| IBIS file stm32u575_585_lqfp100.ibs
[IBIS ver] 4.2
[File name] stm32u575_585_lqfp100.ibs
[File Rev] 1.0
[Date]   06-08-2021
[Source] Data Created at STMicroelectronics
[Notes]  File originated from ELDO simulations.
[Disclaimer]  This information is for modeling purpose only and is
   not guaranted. The information is subject to change without
   notice.
[Copyright] Copyright 2021 STMicroelectronics Inc.
|   Component stm32u575_585_lqfp100
[Component] stm32u575_585_lqfp100
[Manufacturer] STMicroelectronics
[Package]
| variable   typ   min   max
R_pkg   0   NA   NA
L_pkg   0   NA   NA
C_pkg   0   NA   NA
[Pin]   signal_name   model_name   R_pin   L_pin   C_pin   | Comment
1 PE2 io8_100m_hslv_ft 132.430E-3 7.034E-9 135.000E-15
2 PE3 io8_100m_hslv_tamp_ft 133.348E-3 6.765E-9 19.500E-15
3 PE4 io8_100m_hslv_tamp_ft 128.973E-3 6.495E-9 10.400E-15
4 PE5 io8_100m_hslv_tamp_ft 125.345E-3 6.206E-9 5.240E-15
5 PE6 io8_100m_hslv_tamp_ft 120.515E-3 5.991E-9 7.820E-15
6 VBAT POWER 120.471E-3 5.950E-9 6.530E-15
7 PC13 io8_100m_ft_v33 117.881E-3 5.783E-9 6.230E-15
8 PC14-OSC32_IN io8_100m_ft 117.279E-3 5.654E-9 3.110E-15
9 PC15-OSC32_OUT io8_100m_ft 115.548E-3 5.548E-9 1.390E-15
10 VSS GND 114.996E-3 5.434E-9 2.920E-15
11 VDD POWER 112.976E-3 5.296E-9 3.560E-15
12 PH0-OSC_IN io8_100m_ft 111.323E-3 5.231E-9 4.780E-15
13 PH1-OSC_OUT io8_100m_ft 109.217E-3 5.142E-9 8.660E-15
14 NRST nc 110.664E-3 5.180E-9 9.030E-15
15 PC0 io8_100m_hslv_ft 110.608E-3 5.192E-9 7.980E-15
16 PC1 io8_166m_hslv_i2c_ft 111.326E-3 5.252E-9 10.300E-15
17 PC2 io8_100m_hslv_ft 114.420E-3 5.345E-9 7.000E-15
18 PC3 io8_100m_hslv_ft 114.363E-3 5.454E-9 8.650E-15
19 VSSA GND 117.564E-3 5.621E-9 7.825E-15
20 VREF- GND 119.905E-3 5.800E-9 229.000E-18
21 VREF+ POWER 122.312E-3 5.963E-9 1.050E-15
22 VDDA POWER 125.384E-3 6.187E-9 812.000E-18
23 PA0 io8_100m_hslv_tamp_ft 129.702E-3 6.485E-9 3.820E-15
24 PA1 io8_100m_hslv_tamp_ft 132.290E-3 6.715E-9 6.800E-15
25 PA2 io8_100m_hslv_ft 132.955E-3 7.014E-9 16.700E-15
26 PA3 io8_166m_hslv_ft 133.943E-3 7.050E-9 17.500E-15
27 VSS GND 134.958E-3 6.804E-9 12.700E-15
28 VDD POWER 130.511E-3 6.528E-9 9.830E-15
29 PA4 io8_100m_hslv_ft 125.387E-3 6.245E-9 6.070E-15
30 PA5 io8_100m_ft 124.989E-3 6.108E-9 577.000E-18
31 PA6 io8_100m_hslv_ft 121.784E-3 5.890E-9 1.520E-15
32 PA7 io8_100m_hslv_ft 119.149E-3 5.716E-9 5.440E-15
33 PC4 io8_100m_hslv_ft 116.375E-3 5.556E-9 4.100E-15
34 PC5 io8_100m_tamp_ft 113.279E-3 5.415E-9 3.690E-15
35 PB0 io8_100m_hslv_ft 112.727E-3 5.358E-9 3.895E-15
36 PB1 io8_100m_hslv_ft 112.271E-3 5.272E-9 1.660E-15
37 PB2 io8_100m_hslv_tamp_ft 111.816E-3 5.238E-9 7.920E-15
38 PE7 io8_100m_hslv_ft 110.999E-3 5.184E-9 9.900E-15
39 PE8 io8_100m_hslv_ft 114.589E-3 5.299E-9 7.910E-15
40 PE9 io8_166m_hslv_ft 114.461E-3 5.333E-9 7.940E-15
41 PE10 io8_166m_hslv_ft 115.350E-3 5.424E-9 4.180E-15
42 PE11 io8_100m_hslv_ft 116.979E-3 5.533E-9 6.060E-15
43 PE12 io8_100m_hslv_ft 120.185E-3 5.698E-9 5.120E-15
44 PE13 io8_100m_hslv_ft 122.587E-3 5.871E-9 4.740E-15
45 PE14 io8_100m_hslv_ft 126.303E-3 6.069E-9 11.600E-15
46 PE15 io8_100m_hslv_ft 129.715E-3 6.277E-9 9.910E-15
47 PB10 io8_166m_hslv_i2c_ft 133.373E-3 6.508E-9 5.080E-15
48 VCAP POWER 137.888E-3 6.857E-9 5.470E-15
49 VSS GND 131.554E-3 6.802E-9 4.180E-15
50 VDD POWER 132.348E-3 7.042E-9 11.900E-15
51 PB12 io8_166m_hslv_ft 131.768E-3 7.008E-9 16.200E-15
52 PB13 io8_100m_i2c_ft 131.784E-3 6.751E-9 2.150E-15
53 PB14 io8_100m_i2c_ft 129.151E-3 6.483E-9 9.175E-15
54 PB15 nc 125.191E-3 6.202E-9 5.663E-15
55 PD8 io8_100m_hslv_ft 121.530E-3 5.986E-9 3.690E-15
56 PD9 io8_100m_hslv_ft 118.874E-3 5.807E-9 7.430E-15
57 PD10 io8_100m_hslv_ft 115.870E-3 5.635E-9 10.600E-15
58 PD11 io8_100m_hslv_ft 113.226E-3 5.471E-9 5.760E-15
59 PD12 io8_100m_hslv_ft 111.782E-3 5.354E-9 6.530E-15
60 PD13 io8_100m_hslv_ft 110.713E-3 5.276E-9 11.400E-15
61 PD14 io8_100m_hslv_ft 110.052E-3 5.204E-9 13.200E-15
62 PD15 io8_100m_hslv_ft 109.954E-3 5.180E-9 14.600E-15
63 PC6 io8_100m_ft 109.780E-3 5.154E-9 7.250E-15
64 PC7 io8_100m_ft 112.446E-3 5.258E-9 359.000E-18
65 PC8 io8_100m_ft 113.596E-3 5.332E-9 658.000E-18
66 PC9 io8_100m_ft 115.707E-3 5.466E-9 508.500E-18
67 PA8 io8_166m_hslv_ft 116.952E-3 5.598E-9 583.250E-18
68 PA9 io8_100m_usb_vbus_ft 119.043E-3 5.762E-9 545.875E-18
69 PA10 io8_100m_usb_id 120.674E-3 5.880E-9 13.900E-15
70 PA11 io8_usb_ft 124.659E-3 6.108E-9 25.000E-15
71 PA12 io8_usb_ft 124.407E-3 6.161E-9 39.900E-15
72 PA13 io8_100m_ft 130.156E-3 6.404E-9 302.000E-15
73 VDDUSB POWER 135.110E-3 6.824E-9 155.000E-15
74 VSS GND 139.402E-3 7.077E-9 155.000E-15
75 VDD POWER 133.554E-3 7.056E-9 39.000E-15
76 PA14 io8_100m_ft 135.295E-3 7.104E-9 16.300E-15
77 PA15 nc 132.514E-3 6.836E-9 9.760E-15
78 PC10 io8_100m_ft 133.482E-3 6.641E-9 9.300E-15
79 PC11 io8_100m_hslv_ft 128.366E-3 6.341E-9 5.420E-15
80 PC12 io8_166m_hslv_ft 124.282E-3 6.092E-9 1.180E-15
81 PD0 io8_100m_hslv_ft 121.841E-3 5.917E-9 5.460E-15
82 PD1 io8_100m_hslv_ft 118.487E-3 5.728E-9 7.000E-15
83 PD2 io8_100m_ft 117.180E-3 5.573E-9 6.060E-15
84 PD3 io8_166m_hslv_ft 113.501E-3 5.422E-9 5.450E-15
85 PD4 io8_100m_hslv_ft 113.789E-3 5.344E-9 529.000E-18
86 PD5 io8_100m_hslv_ft 110.806E-3 5.256E-9 2.990E-15
87 PD6 io8_166m_hslv_ft 110.442E-3 5.246E-9 2.060E-15
88 PD7 io8_100m_hslv_ft 111.525E-3 5.178E-9 5.680E-15
89 PB3 io8_100m_i2c_ft 111.144E-3 5.223E-9 9.910E-15
90 PB4 io8_100m_i2c_ft 113.222E-3 5.310E-9 9.050E-15
91 PB5 io8_166m_hslv_ft 113.323E-3 5.401E-9 12.900E-15
92 PB6 io8_100m_i2c_ft 115.849E-3 5.519E-9 12.600E-15
93 PB7 io8_166m_hslv_i2c_ft 117.578E-3 5.673E-9 6.140E-15
94 PH3-BOOT0 io8_100m_ft 118.982E-3 5.802E-9 9.370E-15
95 PB8 io8_100m_i2c_ft 121.886E-3 5.962E-9 7.755E-15
96 PB9 io8_100m_i2c_ft 126.276E-3 6.158E-9 8.563E-15
97 PE0 io8_100m_hslv_ft 128.749E-3 6.367E-9 8.159E-15
98 PE1 io8_100m_hslv_ft 133.288E-3 6.700E-9 1.030E-15
99 VSS GND 132.230E-3 6.844E-9 4.410E-15
100 VDD POWER 132.277E-3 7.052E-9 17.100E-15
[Model Selector] io8_100m_ft
io8_100m_ft_hs_1v2  "IO8_FT 100MHz high speed @ 1.2V"
io8_100m_ft_hs_pu_1v2  "IO8_FT 100MHz high speed @ 1.2V pullup"
io8_100m_ft_hs_pd_1v2  "IO8_FT 100MHz high speed @ 1.2V pulldown"
io8_100m_ft_fs_1v2  "IO8_FT 100MHz fast speed @ 1.2V"
io8_100m_ft_fs_pu_1v2  "IO8_FT 100MHz fast speed @ 1.2V pullup"
io8_100m_ft_fs_pd_1v2  "IO8_FT 100MHz fast speed @ 1.2V pulldown"
io8_100m_ft_ms_1v2  "IO8_FT 100MHz med speed @ 1.2V"
io8_100m_ft_ms_pu_1v2  "IO8_FT 100MHz med speed @ 1.2V pullup"
io8_100m_ft_ms_pd_1v2  "IO8_FT 100MHz med speed @ 1.2V pulldown"
io8_100m_ft_ls_1v2  "IO8_FT 100MHz low speed @ 1.2V"
io8_100m_ft_ls_pu_1v2  "IO8_FT 100MHz low speed @ 1.2V pullup"
io8_100m_ft_ls_pd_1v2  "IO8_FT 100MHz low speed @ 1.2V pulldown"
io8_100m_ft_hs_1v8  "IO8_FT 100MHz high speed @ 1.8V"
io8_100m_ft_hs_pu_1v8  "IO8_FT 100MHz high speed @ 1.8V pullup"
io8_100m_ft_hs_pd_1v8  "IO8_FT 100MHz high speed @ 1.8V pulldown"
io8_100m_ft_fs_1v8  "IO8_FT 100MHz fast speed @ 1.8V"
io8_100m_ft_fs_pu_1v8  "IO8_FT 100MHz fast speed @ 1.8V pullup"
io8_100m_ft_fs_pd_1v8  "IO8_FT 100MHz fast speed @ 1.8V pulldown"
io8_100m_ft_ms_1v8  "IO8_FT 100MHz med speed @ 1.8V"
io8_100m_ft_ms_pu_1v8  "IO8_FT 100MHz med speed @ 1.8V pullup"
io8_100m_ft_ms_pd_1v8  "IO8_FT 100MHz med speed @ 1.8V pulldown"
io8_100m_ft_ls_1v8  "IO8_FT 100MHz low speed @ 1.8V"
io8_100m_ft_ls_pu_1v8  "IO8_FT 100MHz low speed @ 1.8V pullup"
io8_100m_ft_ls_pd_1v8  "IO8_FT 100MHz low speed @ 1.8V pulldown"
io8_100m_ft_hs_3v3  "IO8_FT 100MHz high speed @ 3.3V"
io8_100m_ft_hs_pu_3v3  "IO8_FT 100MHz high speed @ 3.3V pullup"
io8_100m_ft_hs_pd_3v3  "IO8_FT 100MHz high speed @ 3.3V pulldown"
io8_100m_ft_fs_3v3  "IO8_FT 100MHz fast speed @ 3.3V"
io8_100m_ft_fs_pu_3v3  "IO8_FT 100MHz fast speed @ 3.3V pullup"
io8_100m_ft_fs_pd_3v3  "IO8_FT 100MHz fast speed @ 3.3V pulldown"
io8_100m_ft_ms_3v3  "IO8_FT 100MHz med speed @ 3.3V"
io8_100m_ft_ms_pu_3v3  "IO8_FT 100MHz med speed @ 3.3V pullup"
io8_100m_ft_ms_pd_3v3  "IO8_FT 100MHz med speed @ 3.3V pulldown"
io8_100m_ft_ls_3v3  "IO8_FT 100MHz low speed @ 3.3V"
io8_100m_ft_ls_pu_3v3  "IO8_FT 100MHz low speed @ 3.3V pullup"
io8_100m_ft_ls_pd_3v3  "IO8_FT 100MHz low speed @ 3.3V pulldown"
[Model Selector] io8_100m_hslv_ft
io8_100m_ft_hs_1v2  "IO8_FT 100MHz high speed @ 1.2V"
io8_100m_ft_hs_pu_1v2  "IO8_FT 100MHz high speed @ 1.2V pullup"
io8_100m_ft_hs_pd_1v2  "IO8_FT 100MHz high speed @ 1.2V pulldown"
io8_100m_ft_fs_1v2  "IO8_FT 100MHz fast speed @ 1.2V"
io8_100m_ft_fs_pu_1v2  "IO8_FT 100MHz fast speed @ 1.2V pullup"
io8_100m_ft_fs_pd_1v2  "IO8_FT 100MHz fast speed @ 1.2V pulldown"
io8_100m_ft_ms_1v2  "IO8_FT 100MHz med speed @ 1.2V"
io8_100m_ft_ms_pu_1v2  "IO8_FT 100MHz med speed @ 1.2V pullup"
io8_100m_ft_ms_pd_1v2  "IO8_FT 100MHz med speed @ 1.2V pulldown"
io8_100m_ft_ls_1v2  "IO8_FT 100MHz low speed @ 1.2V"
io8_100m_ft_ls_pu_1v2  "IO8_FT 100MHz low speed @ 1.2V pullup"
io8_100m_ft_ls_pd_1v2  "IO8_FT 100MHz low speed @ 1.2V pulldown"
io8_100m_ft_hs_1v8  "IO8_FT 100MHz high speed @ 1.8V"
io8_100m_ft_hs_pu_1v8  "IO8_FT 100MHz high speed @ 1.8V pullup"
io8_100m_ft_hs_pd_1v8  "IO8_FT 100MHz high speed @ 1.8V pulldown"
io8_100m_ft_fs_1v8  "IO8_FT 100MHz fast speed @ 1.8V"
io8_100m_ft_fs_pu_1v8  "IO8_FT 100MHz fast speed @ 1.8V pullup"
io8_100m_ft_fs_pd_1v8  "IO8_FT 100MHz fast speed @ 1.8V pulldown"
io8_100m_ft_ms_1v8  "IO8_FT 100MHz med speed @ 1.8V"
io8_100m_ft_ms_pu_1v8  "IO8_FT 100MHz med speed @ 1.8V pullup"
io8_100m_ft_ms_pd_1v8  "IO8_FT 100MHz med speed @ 1.8V pulldown"
io8_100m_ft_ls_1v8  "IO8_FT 100MHz low speed @ 1.8V"
io8_100m_ft_ls_pu_1v8  "IO8_FT 100MHz low speed @ 1.8V pullup"
io8_100m_ft_ls_pd_1v8  "IO8_FT 100MHz low speed @ 1.8V pulldown"
io8_100m_ft_hs_3v3  "IO8_FT 100MHz high speed @ 3.3V"
io8_100m_ft_hs_pu_3v3  "IO8_FT 100MHz high speed @ 3.3V pullup"
io8_100m_ft_hs_pd_3v3  "IO8_FT 100MHz high speed @ 3.3V pulldown"
io8_100m_ft_fs_3v3  "IO8_FT 100MHz fast speed @ 3.3V"
io8_100m_ft_fs_pu_3v3  "IO8_FT 100MHz fast speed @ 3.3V pullup"
io8_100m_ft_fs_pd_3v3  "IO8_FT 100MHz fast speed @ 3.3V pulldown"
io8_100m_ft_ms_3v3  "IO8_FT 100MHz med speed @ 3.3V"
io8_100m_ft_ms_pu_3v3  "IO8_FT 100MHz med speed @ 3.3V pullup"
io8_100m_ft_ms_pd_3v3  "IO8_FT 100MHz med speed @ 3.3V pulldown"
io8_100m_ft_ls_3v3  "IO8_FT 100MHz low speed @ 3.3V"
io8_100m_ft_ls_pu_3v3  "IO8_FT 100MHz low speed @ 3.3V pullup"
io8_100m_ft_ls_pd_3v3  "IO8_FT 100MHz low speed @ 3.3V pulldown"
io8_100m_hslv_ft_hs_1v2  "IO8_FT 100MHz HSLV high speed @ 1.2V"
io8_100m_hslv_ft_hs_pu_1v2  "IO8_FT 100MHz HSLV high speed @ 1.2V pullup"
io8_100m_hslv_ft_hs_pd_1v2  "IO8_FT 100MHz HSLV high speed @ 1.2V pulldown"
io8_100m_hslv_ft_fs_1v2  "IO8_FT 100MHz HSLV fast speed @ 1.2V"
io8_100m_hslv_ft_fs_pu_1v2  "IO8_FT 100MHz HSLV fast speed @ 1.2V pullup"
io8_100m_hslv_ft_fs_pd_1v2  "IO8_FT 100MHz HSLV fast speed @ 1.2V pulldown"
io8_100m_hslv_ft_ms_1v2  "IO8_FT 100MHz HSLV med speed @ 1.2V"
io8_100m_hslv_ft_ms_pu_1v2  "IO8_FT 100MHz HSLV med speed @ 1.2V pullup"
io8_100m_hslv_ft_ms_pd_1v2  "IO8_FT 100MHz HSLV med speed @ 1.2V pulldown"
io8_100m_hslv_ft_ls_1v2  "IO8_FT 100MHz HSLV low speed @ 1.2V"
io8_100m_hslv_ft_ls_pu_1v2  "IO8_FT 100MHz HSLV low speed @ 1.2V pullup"
io8_100m_hslv_ft_ls_pd_1v2  "IO8_FT 100MHz HSLV low speed @ 1.2V pulldown"
io8_100m_hslv_ft_hs_1v8  "IO8_FT 100MHz HSLV high speed @ 1.8V"
io8_100m_hslv_ft_hs_pu_1v8  "IO8_FT 100MHz HSLV high speed @ 1.8V pullup"
io8_100m_hslv_ft_hs_pd_1v8  "IO8_FT 100MHz HSLV high speed @ 1.8V pulldown"
io8_100m_hslv_ft_fs_1v8  "IO8_FT 100MHz HSLV fast speed @ 1.8V"
io8_100m_hslv_ft_fs_pu_1v8  "IO8_FT 100MHz HSLV fast speed @ 1.8V pullup"
io8_100m_hslv_ft_fs_pd_1v8  "IO8_FT 100MHz HSLV fast speed @ 1.8V pulldown"
io8_100m_hslv_ft_ms_1v8  "IO8_FT 100MHz HSLV med speed @ 1.8V"
io8_100m_hslv_ft_ms_pu_1v8  "IO8_FT 100MHz HSLV med speed @ 1.8V pullup"
io8_100m_hslv_ft_ms_pd_1v8  "IO8_FT 100MHz HSLV med speed @ 1.8V pulldown"
io8_100m_hslv_ft_ls_1v8  "IO8_FT 100MHz HSLV low speed @ 1.8V"
io8_100m_hslv_ft_ls_pu_1v8  "IO8_FT 100MHz HSLV low speed @ 1.8V pullup"
io8_100m_hslv_ft_ls_pd_1v8  "IO8_FT 100MHz HSLV low speed @ 1.8V pulldown"
io8_100m_hslv_ft_hs_2v5  "IO8_FT 100MHz HSLV high speed @ 2.5V"
io8_100m_hslv_ft_hs_pu_2v5  "IO8_FT 100MHz HSLV high speed @ 2.5V pullup"
io8_100m_hslv_ft_hs_pd_2v5  "IO8_FT 100MHz HSLV high speed @ 2.5V pulldown"
io8_100m_hslv_ft_fs_2v5  "IO8_FT 100MHz HSLV fast speed @ 2.5V"
io8_100m_hslv_ft_fs_pu_2v5  "IO8_FT 100MHz HSLV fast speed @ 2.5V pullup"
io8_100m_hslv_ft_fs_pd_2v5  "IO8_FT 100MHz HSLV fast speed @ 2.5V pulldown"
io8_100m_hslv_ft_ms_2v5  "IO8_FT 100MHz HSLV med speed @ 2.5V"
io8_100m_hslv_ft_ms_pu_2v5  "IO8_FT 100MHz HSLV med speed @ 2.5V pullup"
io8_100m_hslv_ft_ms_pd_2v5  "IO8_FT 100MHz HSLV med speed @ 2.5V pulldown"
io8_100m_hslv_ft_ls_2v5  "IO8_FT 100MHz HSLV low speed @ 2.5V"
io8_100m_hslv_ft_ls_pu_2v5  "IO8_FT 100MHz HSLV low speed @ 2.5V pullup"
io8_100m_hslv_ft_ls_pd_2v5  "IO8_FT 100MHz HSLV low speed @ 2.5V pulldown"
[Model Selector] io8_166m_hslv_ft
io8_166m_ft_hs_1v2  "IO8_FT 166MHz high speed @ 1.2V"
io8_166m_ft_hs_pu_1v2  "IO8_FT 166MHz high speed @ 1.2V pullup"
io8_166m_ft_hs_pd_1v2  "IO8_FT 166MHz high speed @ 1.2V pulldown"
io8_166m_ft_fs_1v2  "IO8_FT 166MHz fast speed @ 1.2V"
io8_166m_ft_fs_pu_1v2  "IO8_FT 166MHz fast speed @ 1.2V pullup"
io8_166m_ft_fs_pd_1v2  "IO8_FT 166MHz fast speed @ 1.2V pulldown"
io8_166m_ft_ms_1v2  "IO8_FT 166MHz med speed @ 1.2V"
io8_166m_ft_ms_pu_1v2  "IO8_FT 166MHz med speed @ 1.2V pullup"
io8_166m_ft_ms_pd_1v2  "IO8_FT 166MHz med speed @ 1.2V pulldown"
io8_166m_ft_ls_1v2  "IO8_FT 166MHz low speed @ 1.2V"
io8_166m_ft_ls_pu_1v2  "IO8_FT 166MHz low speed @ 1.2V pullup"
io8_166m_ft_ls_pd_1v2  "IO8_FT 166MHz low speed @ 1.2V pulldown"
io8_166m_ft_hs_1v8  "IO8_FT 166MHz high speed @ 1.8V"
io8_166m_ft_hs_pu_1v8  "IO8_FT 166MHz high speed @ 1.8V pullup"
io8_166m_ft_hs_pd_1v8  "IO8_FT 166MHz high speed @ 1.8V pulldown"
io8_166m_ft_fs_1v8  "IO8_FT 166MHz fast speed @ 1.8V"
io8_166m_ft_fs_pu_1v8  "IO8_FT 166MHz fast speed @ 1.8V pullup"
io8_166m_ft_fs_pd_1v8  "IO8_FT 166MHz fast speed @ 1.8V pulldown"
io8_166m_ft_ms_1v8  "IO8_FT 166MHz med speed @ 1.8V"
io8_166m_ft_ms_pu_1v8  "IO8_FT 166MHz med speed @ 1.8V pullup"
io8_166m_ft_ms_pd_1v8  "IO8_FT 166MHz med speed @ 1.8V pulldown"
io8_166m_ft_ls_1v8  "IO8_FT 166MHz low speed @ 1.8V"
io8_166m_ft_ls_pu_1v8  "IO8_FT 166MHz low speed @ 1.8V pullup"
io8_166m_ft_ls_pd_1v8  "IO8_FT 166MHz low speed @ 1.8V pulldown"
io8_166m_ft_hs_3v3  "IO8_FT 166MHz high speed @ 3.3V"
io8_166m_ft_hs_pu_3v3  "IO8_FT 166MHz high speed @ 3.3V pullup"
io8_166m_ft_hs_pd_3v3  "IO8_FT 166MHz high speed @ 3.3V pulldown"
io8_166m_ft_fs_3v3  "IO8_FT 166MHz fast speed @ 3.3V"
io8_166m_ft_fs_pu_3v3  "IO8_FT 166MHz fast speed @ 3.3V pullup"
io8_166m_ft_fs_pd_3v3  "IO8_FT 166MHz fast speed @ 3.3V pulldown"
io8_166m_ft_ms_3v3  "IO8_FT 166MHz med speed @ 3.3V"
io8_166m_ft_ms_pu_3v3  "IO8_FT 166MHz med speed @ 3.3V pullup"
io8_166m_ft_ms_pd_3v3  "IO8_FT 166MHz med speed @ 3.3V pulldown"
io8_166m_ft_ls_3v3  "IO8_FT 166MHz low speed @ 3.3V"
io8_166m_ft_ls_pu_3v3  "IO8_FT 166MHz low speed @ 3.3V pullup"
io8_166m_ft_ls_pd_3v3  "IO8_FT 166MHz low speed @ 3.3V pulldown"
io8_166m_hslv_ft_hs_1v2  "IO8_FT 166MHz HSLV high speed @ 1.2V"
io8_166m_hslv_ft_hs_pu_1v2  "IO8_FT 166MHz HSLV high speed @ 1.2V pullup"
io8_166m_hslv_ft_hs_pd_1v2  "IO8_FT 166MHz HSLV high speed @ 1.2V pulldown"
io8_166m_hslv_ft_fs_1v2  "IO8_FT 166MHz HSLV fast speed @ 1.2V"
io8_166m_hslv_ft_fs_pu_1v2  "IO8_FT 166MHz HSLV fast speed @ 1.2V pullup"
io8_166m_hslv_ft_fs_pd_1v2  "IO8_FT 166MHz HSLV fast speed @ 1.2V pulldown"
io8_166m_hslv_ft_ms_1v2  "IO8_FT 166MHz HSLV med speed @ 1.2V"
io8_166m_hslv_ft_ms_pu_1v2  "IO8_FT 166MHz HSLV med speed @ 1.2V pullup"
io8_166m_hslv_ft_ms_pd_1v2  "IO8_FT 166MHz HSLV med speed @ 1.2V pulldown"
io8_166m_hslv_ft_ls_1v2  "IO8_FT 166MHz HSLV low speed @ 1.2V"
io8_166m_hslv_ft_ls_pu_1v2  "IO8_FT 166MHz HSLV low speed @ 1.2V pullup"
io8_166m_hslv_ft_ls_pd_1v2  "IO8_FT 166MHz HSLV low speed @ 1.2V pulldown"
io8_166m_hslv_ft_hs_1v8  "IO8_FT 166MHz HSLV high speed @ 1.8V"
io8_166m_hslv_ft_hs_pu_1v8  "IO8_FT 166MHz HSLV high speed @ 1.8V pullup"
io8_166m_hslv_ft_hs_pd_1v8  "IO8_FT 166MHz HSLV high speed @ 1.8V pulldown"
io8_166m_hslv_ft_fs_1v8  "IO8_FT 166MHz HSLV fast speed @ 1.8V"
io8_166m_hslv_ft_fs_pu_1v8  "IO8_FT 166MHz HSLV fast speed @ 1.8V pullup"
io8_166m_hslv_ft_fs_pd_1v8  "IO8_FT 166MHz HSLV fast speed @ 1.8V pulldown"
io8_166m_hslv_ft_ms_1v8  "IO8_FT 166MHz HSLV med speed @ 1.8V"
io8_166m_hslv_ft_ms_pu_1v8  "IO8_FT 166MHz HSLV med speed @ 1.8V pullup"
io8_166m_hslv_ft_ms_pd_1v8  "IO8_FT 166MHz HSLV med speed @ 1.8V pulldown"
io8_166m_hslv_ft_ls_1v8  "IO8_FT 166MHz HSLV low speed @ 1.8V"
io8_166m_hslv_ft_ls_pu_1v8  "IO8_FT 166MHz HSLV low speed @ 1.8V pullup"
io8_166m_hslv_ft_ls_pd_1v8  "IO8_FT 166MHz HSLV low speed @ 1.8V pulldown"
io8_166m_hslv_ft_hs_2v5  "IO8_FT 166MHz HSLV high speed @ 2.5V"
io8_166m_hslv_ft_hs_pu_2v5  "IO8_FT 166MHz HSLV high speed @ 2.5V pullup"
io8_166m_hslv_ft_hs_pd_2v5  "IO8_FT 166MHz HSLV high speed @ 2.5V pulldown"
io8_166m_hslv_ft_fs_2v5  "IO8_FT 166MHz HSLV fast speed @ 2.5V"
io8_166m_hslv_ft_fs_pu_2v5  "IO8_FT 166MHz HSLV fast speed @ 2.5V pullup"
io8_166m_hslv_ft_fs_pd_2v5  "IO8_FT 166MHz HSLV fast speed @ 2.5V pulldown"
io8_166m_hslv_ft_ms_2v5  "IO8_FT 166MHz HSLV med speed @ 2.5V"
io8_166m_hslv_ft_ms_pu_2v5  "IO8_FT 166MHz HSLV med speed @ 2.5V pullup"
io8_166m_hslv_ft_ms_pd_2v5  "IO8_FT 166MHz HSLV med speed @ 2.5V pulldown"
io8_166m_hslv_ft_ls_2v5  "IO8_FT 166MHz HSLV low speed @ 2.5V"
io8_166m_hslv_ft_ls_pu_2v5  "IO8_FT 166MHz HSLV low speed @ 2.5V pullup"
io8_166m_hslv_ft_ls_pd_2v5  "IO8_FT 166MHz HSLV low speed @ 2.5V pulldown"
[Model Selector] io8_100m_ft_v33
io8_ft_v33_hs_1v2  "IO8_FT_V33 high speed @ 1.2V"
io8_ft_v33_hs_pu_1v2  "IO8_FT_V33 high speed @ 1.2V pullup"
io8_ft_v33_hs_pd_1v2  "IO8_FT_V33 high speed @ 1.2V pulldown"
io8_ft_v33_fs_1v2  "IO8_FT_V33 fast speed @ 1.2V"
io8_ft_v33_fs_pu_1v2  "IO8_FT_V33 fast speed @ 1.2V pullup"
io8_ft_v33_fs_pd_1v2  "IO8_FT_V33 fast speed @ 1.2V pulldown"
io8_ft_v33_ms_1v2  "IO8_FT_V33 med speed @ 1.2V"
io8_ft_v33_ms_pu_1v2  "IO8_FT_V33 med speed @ 1.2V pullup"
io8_ft_v33_ms_pd_1v2  "IO8_FT_V33 med speed @ 1.2V pulldown"
io8_ft_v33_ls_1v2  "IO8_FT_V33 low speed @ 1.2V"
io8_ft_v33_ls_pu_1v2  "IO8_FT_V33 low speed @ 1.2V pullup"
io8_ft_v33_ls_pd_1v2  "IO8_FT_V33 low speed @ 1.2V pulldown"
io8_ft_v33_hs_1v8  "IO8_FT_V33 high speed @ 1.8V"
io8_ft_v33_hs_pu_1v8  "IO8_FT_V33 high speed @ 1.8V pullup"
io8_ft_v33_hs_pd_1v8  "IO8_FT_V33 high speed @ 1.8V pulldown"
io8_ft_v33_fs_1v8  "IO8_FT_V33 fast speed @ 1.8V"
io8_ft_v33_fs_pu_1v8  "IO8_FT_V33 fast speed @ 1.8V pullup"
io8_ft_v33_fs_pd_1v8  "IO8_FT_V33 fast speed @ 1.8V pulldown"
io8_ft_v33_ms_1v8  "IO8_FT_V33 med speed @ 1.8V"
io8_ft_v33_ms_pu_1v8  "IO8_FT_V33 med speed @ 1.8V pullup"
io8_ft_v33_ms_pd_1v8  "IO8_FT_V33 med speed @ 1.8V pulldown"
io8_ft_v33_ls_1v8  "IO8_FT_V33 low speed @ 1.8V"
io8_ft_v33_ls_pu_1v8  "IO8_FT_V33 low speed @ 1.8V pullup"
io8_ft_v33_ls_pd_1v8  "IO8_FT_V33 low speed @ 1.8V pulldown"
io8_ft_v33_hs_3v3  "IO8_FT_V33 high speed @ 3.3V"
io8_ft_v33_hs_pu_3v3  "IO8_FT_V33 high speed @ 3.3V pullup"
io8_ft_v33_hs_pd_3v3  "IO8_FT_V33 high speed @ 3.3V pulldown"
io8_ft_v33_fs_3v3  "IO8_FT_V33 fast speed @ 3.3V"
io8_ft_v33_fs_pu_3v3  "IO8_FT_V33 fast speed @ 3.3V pullup"
io8_ft_v33_fs_pd_3v3  "IO8_FT_V33 fast speed @ 3.3V pulldown"
io8_ft_v33_ms_3v3  "IO8_FT_V33 med speed @ 3.3V"
io8_ft_v33_ms_pu_3v3  "IO8_FT_V33 med speed @ 3.3V pullup"
io8_ft_v33_ms_pd_3v3  "IO8_FT_V33 med speed @ 3.3V pulldown"
io8_ft_v33_ls_3v3  "IO8_FT_V33 low speed @ 3.3V"
io8_ft_v33_ls_pu_3v3  "IO8_FT_V33 low speed @ 3.3V pullup"
io8_ft_v33_ls_pd_3v3  "IO8_FT_V33 low speed @ 3.3V pulldown"
[Model Selector] io8_100m_tamp_ft
io8_100m_ft_hs_1v2  "IO8_FT 100MHz high speed @ 1.2V"
io8_100m_ft_hs_pu_1v2  "IO8_FT 100MHz high speed @ 1.2V pullup"
io8_100m_ft_hs_pd_1v2  "IO8_FT 100MHz high speed @ 1.2V pulldown"
io8_100m_ft_fs_1v2  "IO8_FT 100MHz fast speed @ 1.2V"
io8_100m_ft_fs_pu_1v2  "IO8_FT 100MHz fast speed @ 1.2V pullup"
io8_100m_ft_fs_pd_1v2  "IO8_FT 100MHz fast speed @ 1.2V pulldown"
io8_100m_ft_ms_1v2  "IO8_FT 100MHz med speed @ 1.2V"
io8_100m_ft_ms_pu_1v2  "IO8_FT 100MHz med speed @ 1.2V pullup"
io8_100m_ft_ms_pd_1v2  "IO8_FT 100MHz med speed @ 1.2V pulldown"
io8_100m_ft_ls_1v2  "IO8_FT 100MHz low speed @ 1.2V"
io8_100m_ft_ls_pu_1v2  "IO8_FT 100MHz low speed @ 1.2V pullup"
io8_100m_ft_ls_pd_1v2  "IO8_FT 100MHz low speed @ 1.2V pulldown"
io8_100m_ft_hs_1v8  "IO8_FT 100MHz high speed @ 1.8V"
io8_100m_ft_hs_pu_1v8  "IO8_FT 100MHz high speed @ 1.8V pullup"
io8_100m_ft_hs_pd_1v8  "IO8_FT 100MHz high speed @ 1.8V pulldown"
io8_100m_ft_fs_1v8  "IO8_FT 100MHz fast speed @ 1.8V"
io8_100m_ft_fs_pu_1v8  "IO8_FT 100MHz fast speed @ 1.8V pullup"
io8_100m_ft_fs_pd_1v8  "IO8_FT 100MHz fast speed @ 1.8V pulldown"
io8_100m_ft_ms_1v8  "IO8_FT 100MHz med speed @ 1.8V"
io8_100m_ft_ms_pu_1v8  "IO8_FT 100MHz med speed @ 1.8V pullup"
io8_100m_ft_ms_pd_1v8  "IO8_FT 100MHz med speed @ 1.8V pulldown"
io8_100m_ft_ls_1v8  "IO8_FT 100MHz low speed @ 1.8V"
io8_100m_ft_ls_pu_1v8  "IO8_FT 100MHz low speed @ 1.8V pullup"
io8_100m_ft_ls_pd_1v8  "IO8_FT 100MHz low speed @ 1.8V pulldown"
io8_100m_ft_hs_3v3  "IO8_FT 100MHz high speed @ 3.3V"
io8_100m_ft_hs_pu_3v3  "IO8_FT 100MHz high speed @ 3.3V pullup"
io8_100m_ft_hs_pd_3v3  "IO8_FT 100MHz high speed @ 3.3V pulldown"
io8_100m_ft_fs_3v3  "IO8_FT 100MHz fast speed @ 3.3V"
io8_100m_ft_fs_pu_3v3  "IO8_FT 100MHz fast speed @ 3.3V pullup"
io8_100m_ft_fs_pd_3v3  "IO8_FT 100MHz fast speed @ 3.3V pulldown"
io8_100m_ft_ms_3v3  "IO8_FT 100MHz med speed @ 3.3V"
io8_100m_ft_ms_pu_3v3  "IO8_FT 100MHz med speed @ 3.3V pullup"
io8_100m_ft_ms_pd_3v3  "IO8_FT 100MHz med speed @ 3.3V pulldown"
io8_100m_ft_ls_3v3  "IO8_FT 100MHz low speed @ 3.3V"
io8_100m_ft_ls_pu_3v3  "IO8_FT 100MHz low speed @ 3.3V pullup"
io8_100m_ft_ls_pd_3v3  "IO8_FT 100MHz low speed @ 3.3V pulldown"
io8_ft_v33_hs_1v2  "IO8_FT_V33 high speed @ 1.2V"
io8_ft_v33_hs_pu_1v2  "IO8_FT_V33 high speed @ 1.2V pullup"
io8_ft_v33_hs_pd_1v2  "IO8_FT_V33 high speed @ 1.2V pulldown"
io8_ft_v33_fs_1v2  "IO8_FT_V33 fast speed @ 1.2V"
io8_ft_v33_fs_pu_1v2  "IO8_FT_V33 fast speed @ 1.2V pullup"
io8_ft_v33_fs_pd_1v2  "IO8_FT_V33 fast speed @ 1.2V pulldown"
io8_ft_v33_ms_1v2  "IO8_FT_V33 med speed @ 1.2V"
io8_ft_v33_ms_pu_1v2  "IO8_FT_V33 med speed @ 1.2V pullup"
io8_ft_v33_ms_pd_1v2  "IO8_FT_V33 med speed @ 1.2V pulldown"
io8_ft_v33_ls_1v2  "IO8_FT_V33 low speed @ 1.2V"
io8_ft_v33_ls_pu_1v2  "IO8_FT_V33 low speed @ 1.2V pullup"
io8_ft_v33_ls_pd_1v2  "IO8_FT_V33 low speed @ 1.2V pulldown"
io8_ft_v33_hs_1v8  "IO8_FT_V33 high speed @ 1.8V"
io8_ft_v33_hs_pu_1v8  "IO8_FT_V33 high speed @ 1.8V pullup"
io8_ft_v33_hs_pd_1v8  "IO8_FT_V33 high speed @ 1.8V pulldown"
io8_ft_v33_fs_1v8  "IO8_FT_V33 fast speed @ 1.8V"
io8_ft_v33_fs_pu_1v8  "IO8_FT_V33 fast speed @ 1.8V pullup"
io8_ft_v33_fs_pd_1v8  "IO8_FT_V33 fast speed @ 1.8V pulldown"
io8_ft_v33_ms_1v8  "IO8_FT_V33 med speed @ 1.8V"
io8_ft_v33_ms_pu_1v8  "IO8_FT_V33 med speed @ 1.8V pullup"
io8_ft_v33_ms_pd_1v8  "IO8_FT_V33 med speed @ 1.8V pulldown"
io8_ft_v33_ls_1v8  "IO8_FT_V33 low speed @ 1.8V"
io8_ft_v33_ls_pu_1v8  "IO8_FT_V33 low speed @ 1.8V pullup"
io8_ft_v33_ls_pd_1v8  "IO8_FT_V33 low speed @ 1.8V pulldown"
io8_ft_v33_hs_3v3  "IO8_FT_V33 high speed @ 3.3V"
io8_ft_v33_hs_pu_3v3  "IO8_FT_V33 high speed @ 3.3V pullup"
io8_ft_v33_hs_pd_3v3  "IO8_FT_V33 high speed @ 3.3V pulldown"
io8_ft_v33_fs_3v3  "IO8_FT_V33 fast speed @ 3.3V"
io8_ft_v33_fs_pu_3v3  "IO8_FT_V33 fast speed @ 3.3V pullup"
io8_ft_v33_fs_pd_3v3  "IO8_FT_V33 fast speed @ 3.3V pulldown"
io8_ft_v33_ms_3v3  "IO8_FT_V33 med speed @ 3.3V"
io8_ft_v33_ms_pu_3v3  "IO8_FT_V33 med speed @ 3.3V pullup"
io8_ft_v33_ms_pd_3v3  "IO8_FT_V33 med speed @ 3.3V pulldown"
io8_ft_v33_ls_3v3  "IO8_FT_V33 low speed @ 3.3V"
io8_ft_v33_ls_pu_3v3  "IO8_FT_V33 low speed @ 3.3V pullup"
io8_ft_v33_ls_pd_3v3  "IO8_FT_V33 low speed @ 3.3V pulldown"
[Model Selector] io8_100m_hslv_tamp_ft
io8_100m_ft_hs_1v2  "IO8_FT 100MHz high speed @ 1.2V"
io8_100m_ft_hs_pu_1v2  "IO8_FT 100MHz high speed @ 1.2V pullup"
io8_100m_ft_hs_pd_1v2  "IO8_FT 100MHz high speed @ 1.2V pulldown"
io8_100m_ft_fs_1v2  "IO8_FT 100MHz fast speed @ 1.2V"
io8_100m_ft_fs_pu_1v2  "IO8_FT 100MHz fast speed @ 1.2V pullup"
io8_100m_ft_fs_pd_1v2  "IO8_FT 100MHz fast speed @ 1.2V pulldown"
io8_100m_ft_ms_1v2  "IO8_FT 100MHz med speed @ 1.2V"
io8_100m_ft_ms_pu_1v2  "IO8_FT 100MHz med speed @ 1.2V pullup"
io8_100m_ft_ms_pd_1v2  "IO8_FT 100MHz med speed @ 1.2V pulldown"
io8_100m_ft_ls_1v2  "IO8_FT 100MHz low speed @ 1.2V"
io8_100m_ft_ls_pu_1v2  "IO8_FT 100MHz low speed @ 1.2V pullup"
io8_100m_ft_ls_pd_1v2  "IO8_FT 100MHz low speed @ 1.2V pulldown"
io8_100m_ft_hs_1v8  "IO8_FT 100MHz high speed @ 1.8V"
io8_100m_ft_hs_pu_1v8  "IO8_FT 100MHz high speed @ 1.8V pullup"
io8_100m_ft_hs_pd_1v8  "IO8_FT 100MHz high speed @ 1.8V pulldown"
io8_100m_ft_fs_1v8  "IO8_FT 100MHz fast speed @ 1.8V"
io8_100m_ft_fs_pu_1v8  "IO8_FT 100MHz fast speed @ 1.8V pullup"
io8_100m_ft_fs_pd_1v8  "IO8_FT 100MHz fast speed @ 1.8V pulldown"
io8_100m_ft_ms_1v8  "IO8_FT 100MHz med speed @ 1.8V"
io8_100m_ft_ms_pu_1v8  "IO8_FT 100MHz med speed @ 1.8V pullup"
io8_100m_ft_ms_pd_1v8  "IO8_FT 100MHz med speed @ 1.8V pulldown"
io8_100m_ft_ls_1v8  "IO8_FT 100MHz low speed @ 1.8V"
io8_100m_ft_ls_pu_1v8  "IO8_FT 100MHz low speed @ 1.8V pullup"
io8_100m_ft_ls_pd_1v8  "IO8_FT 100MHz low speed @ 1.8V pulldown"
io8_100m_ft_hs_3v3  "IO8_FT 100MHz high speed @ 3.3V"
io8_100m_ft_hs_pu_3v3  "IO8_FT 100MHz high speed @ 3.3V pullup"
io8_100m_ft_hs_pd_3v3  "IO8_FT 100MHz high speed @ 3.3V pulldown"
io8_100m_ft_fs_3v3  "IO8_FT 100MHz fast speed @ 3.3V"
io8_100m_ft_fs_pu_3v3  "IO8_FT 100MHz fast speed @ 3.3V pullup"
io8_100m_ft_fs_pd_3v3  "IO8_FT 100MHz fast speed @ 3.3V pulldown"
io8_100m_ft_ms_3v3  "IO8_FT 100MHz med speed @ 3.3V"
io8_100m_ft_ms_pu_3v3  "IO8_FT 100MHz med speed @ 3.3V pullup"
io8_100m_ft_ms_pd_3v3  "IO8_FT 100MHz med speed @ 3.3V pulldown"
io8_100m_ft_ls_3v3  "IO8_FT 100MHz low speed @ 3.3V"
io8_100m_ft_ls_pu_3v3  "IO8_FT 100MHz low speed @ 3.3V pullup"
io8_100m_ft_ls_pd_3v3  "IO8_FT 100MHz low speed @ 3.3V pulldown"
io8_100m_hslv_ft_hs_1v2  "IO8_FT 100MHz HSLV high speed @ 1.2V"
io8_100m_hslv_ft_hs_pu_1v2  "IO8_FT 100MHz HSLV high speed @ 1.2V pullup"
io8_100m_hslv_ft_hs_pd_1v2  "IO8_FT 100MHz HSLV high speed @ 1.2V pulldown"
io8_100m_hslv_ft_fs_1v2  "IO8_FT 100MHz HSLV fast speed @ 1.2V"
io8_100m_hslv_ft_fs_pu_1v2  "IO8_FT 100MHz HSLV fast speed @ 1.2V pullup"
io8_100m_hslv_ft_fs_pd_1v2  "IO8_FT 100MHz HSLV fast speed @ 1.2V pulldown"
io8_100m_hslv_ft_ms_1v2  "IO8_FT 100MHz HSLV med speed @ 1.2V"
io8_100m_hslv_ft_ms_pu_1v2  "IO8_FT 100MHz HSLV med speed @ 1.2V pullup"
io8_100m_hslv_ft_ms_pd_1v2  "IO8_FT 100MHz HSLV med speed @ 1.2V pulldown"
io8_100m_hslv_ft_ls_1v2  "IO8_FT 100MHz HSLV low speed @ 1.2V"
io8_100m_hslv_ft_ls_pu_1v2  "IO8_FT 100MHz HSLV low speed @ 1.2V pullup"
io8_100m_hslv_ft_ls_pd_1v2  "IO8_FT 100MHz HSLV low speed @ 1.2V pulldown"
io8_100m_hslv_ft_hs_1v8  "IO8_FT 100MHz HSLV high speed @ 1.8V"
io8_100m_hslv_ft_hs_pu_1v8  "IO8_FT 100MHz HSLV high speed @ 1.8V pullup"
io8_100m_hslv_ft_hs_pd_1v8  "IO8_FT 100MHz HSLV high speed @ 1.8V pulldown"
io8_100m_hslv_ft_fs_1v8  "IO8_FT 100MHz HSLV fast speed @ 1.8V"
io8_100m_hslv_ft_fs_pu_1v8  "IO8_FT 100MHz HSLV fast speed @ 1.8V pullup"
io8_100m_hslv_ft_fs_pd_1v8  "IO8_FT 100MHz HSLV fast speed @ 1.8V pulldown"
io8_100m_hslv_ft_ms_1v8  "IO8_FT 100MHz HSLV med speed @ 1.8V"
io8_100m_hslv_ft_ms_pu_1v8  "IO8_FT 100MHz HSLV med speed @ 1.8V pullup"
io8_100m_hslv_ft_ms_pd_1v8  "IO8_FT 100MHz HSLV med speed @ 1.8V pulldown"
io8_100m_hslv_ft_ls_1v8  "IO8_FT 100MHz HSLV low speed @ 1.8V"
io8_100m_hslv_ft_ls_pu_1v8  "IO8_FT 100MHz HSLV low speed @ 1.8V pullup"
io8_100m_hslv_ft_ls_pd_1v8  "IO8_FT 100MHz HSLV low speed @ 1.8V pulldown"
io8_100m_hslv_ft_hs_2v5  "IO8_FT 100MHz HSLV high speed @ 2.5V"
io8_100m_hslv_ft_hs_pu_2v5  "IO8_FT 100MHz HSLV high speed @ 2.5V pullup"
io8_100m_hslv_ft_hs_pd_2v5  "IO8_FT 100MHz HSLV high speed @ 2.5V pulldown"
io8_100m_hslv_ft_fs_2v5  "IO8_FT 100MHz HSLV fast speed @ 2.5V"
io8_100m_hslv_ft_fs_pu_2v5  "IO8_FT 100MHz HSLV fast speed @ 2.5V pullup"
io8_100m_hslv_ft_fs_pd_2v5  "IO8_FT 100MHz HSLV fast speed @ 2.5V pulldown"
io8_100m_hslv_ft_ms_2v5  "IO8_FT 100MHz HSLV med speed @ 2.5V"
io8_100m_hslv_ft_ms_pu_2v5  "IO8_FT 100MHz HSLV med speed @ 2.5V pullup"
io8_100m_hslv_ft_ms_pd_2v5  "IO8_FT 100MHz HSLV med speed @ 2.5V pulldown"
io8_100m_hslv_ft_ls_2v5  "IO8_FT 100MHz HSLV low speed @ 2.5V"
io8_100m_hslv_ft_ls_pu_2v5  "IO8_FT 100MHz HSLV low speed @ 2.5V pullup"
io8_100m_hslv_ft_ls_pd_2v5  "IO8_FT 100MHz HSLV low speed @ 2.5V pulldown"
io8_ft_v33_hs_1v2  "IO8_FT_V33 high speed @ 1.2V"
io8_ft_v33_hs_pu_1v2  "IO8_FT_V33 high speed @ 1.2V pullup"
io8_ft_v33_hs_pd_1v2  "IO8_FT_V33 high speed @ 1.2V pulldown"
io8_ft_v33_fs_1v2  "IO8_FT_V33 fast speed @ 1.2V"
io8_ft_v33_fs_pu_1v2  "IO8_FT_V33 fast speed @ 1.2V pullup"
io8_ft_v33_fs_pd_1v2  "IO8_FT_V33 fast speed @ 1.2V pulldown"
io8_ft_v33_ms_1v2  "IO8_FT_V33 med speed @ 1.2V"
io8_ft_v33_ms_pu_1v2  "IO8_FT_V33 med speed @ 1.2V pullup"
io8_ft_v33_ms_pd_1v2  "IO8_FT_V33 med speed @ 1.2V pulldown"
io8_ft_v33_ls_1v2  "IO8_FT_V33 low speed @ 1.2V"
io8_ft_v33_ls_pu_1v2  "IO8_FT_V33 low speed @ 1.2V pullup"
io8_ft_v33_ls_pd_1v2  "IO8_FT_V33 low speed @ 1.2V pulldown"
io8_ft_v33_hs_1v8  "IO8_FT_V33 high speed @ 1.8V"
io8_ft_v33_hs_pu_1v8  "IO8_FT_V33 high speed @ 1.8V pullup"
io8_ft_v33_hs_pd_1v8  "IO8_FT_V33 high speed @ 1.8V pulldown"
io8_ft_v33_fs_1v8  "IO8_FT_V33 fast speed @ 1.8V"
io8_ft_v33_fs_pu_1v8  "IO8_FT_V33 fast speed @ 1.8V pullup"
io8_ft_v33_fs_pd_1v8  "IO8_FT_V33 fast speed @ 1.8V pulldown"
io8_ft_v33_ms_1v8  "IO8_FT_V33 med speed @ 1.8V"
io8_ft_v33_ms_pu_1v8  "IO8_FT_V33 med speed @ 1.8V pullup"
io8_ft_v33_ms_pd_1v8  "IO8_FT_V33 med speed @ 1.8V pulldown"
io8_ft_v33_ls_1v8  "IO8_FT_V33 low speed @ 1.8V"
io8_ft_v33_ls_pu_1v8  "IO8_FT_V33 low speed @ 1.8V pullup"
io8_ft_v33_ls_pd_1v8  "IO8_FT_V33 low speed @ 1.8V pulldown"
io8_ft_v33_hs_3v3  "IO8_FT_V33 high speed @ 3.3V"
io8_ft_v33_hs_pu_3v3  "IO8_FT_V33 high speed @ 3.3V pullup"
io8_ft_v33_hs_pd_3v3  "IO8_FT_V33 high speed @ 3.3V pulldown"
io8_ft_v33_fs_3v3  "IO8_FT_V33 fast speed @ 3.3V"
io8_ft_v33_fs_pu_3v3  "IO8_FT_V33 fast speed @ 3.3V pullup"
io8_ft_v33_fs_pd_3v3  "IO8_FT_V33 fast speed @ 3.3V pulldown"
io8_ft_v33_ms_3v3  "IO8_FT_V33 med speed @ 3.3V"
io8_ft_v33_ms_pu_3v3  "IO8_FT_V33 med speed @ 3.3V pullup"
io8_ft_v33_ms_pd_3v3  "IO8_FT_V33 med speed @ 3.3V pulldown"
io8_ft_v33_ls_3v3  "IO8_FT_V33 low speed @ 3.3V"
io8_ft_v33_ls_pu_3v3  "IO8_FT_V33 low speed @ 3.3V pullup"
io8_ft_v33_ls_pd_3v3  "IO8_FT_V33 low speed @ 3.3V pulldown"
[Model Selector] io8_100m_usb_id
io8_100m_ft_hs_1v2  "IO8_FT 100MHz high speed @ 1.2V"
io8_100m_ft_hs_pu_1v2  "IO8_FT 100MHz high speed @ 1.2V pullup"
io8_100m_ft_hs_pd_1v2  "IO8_FT 100MHz high speed @ 1.2V pulldown"
io8_100m_ft_fs_1v2  "IO8_FT 100MHz fast speed @ 1.2V"
io8_100m_ft_fs_pu_1v2  "IO8_FT 100MHz fast speed @ 1.2V pullup"
io8_100m_ft_fs_pd_1v2  "IO8_FT 100MHz fast speed @ 1.2V pulldown"
io8_100m_ft_ms_1v2  "IO8_FT 100MHz med speed @ 1.2V"
io8_100m_ft_ms_pu_1v2  "IO8_FT 100MHz med speed @ 1.2V pullup"
io8_100m_ft_ms_pd_1v2  "IO8_FT 100MHz med speed @ 1.2V pulldown"
io8_100m_ft_ls_1v2  "IO8_FT 100MHz low speed @ 1.2V"
io8_100m_ft_ls_pu_1v2  "IO8_FT 100MHz low speed @ 1.2V pullup"
io8_100m_ft_ls_pd_1v2  "IO8_FT 100MHz low speed @ 1.2V pulldown"
io8_100m_ft_hs_1v8  "IO8_FT 100MHz high speed @ 1.8V"
io8_100m_ft_hs_pu_1v8  "IO8_FT 100MHz high speed @ 1.8V pullup"
io8_100m_ft_hs_pd_1v8  "IO8_FT 100MHz high speed @ 1.8V pulldown"
io8_100m_ft_fs_1v8  "IO8_FT 100MHz fast speed @ 1.8V"
io8_100m_ft_fs_pu_1v8  "IO8_FT 100MHz fast speed @ 1.8V pullup"
io8_100m_ft_fs_pd_1v8  "IO8_FT 100MHz fast speed @ 1.8V pulldown"
io8_100m_ft_ms_1v8  "IO8_FT 100MHz med speed @ 1.8V"
io8_100m_ft_ms_pu_1v8  "IO8_FT 100MHz med speed @ 1.8V pullup"
io8_100m_ft_ms_pd_1v8  "IO8_FT 100MHz med speed @ 1.8V pulldown"
io8_100m_ft_ls_1v8  "IO8_FT 100MHz low speed @ 1.8V"
io8_100m_ft_ls_pu_1v8  "IO8_FT 100MHz low speed @ 1.8V pullup"
io8_100m_ft_ls_pd_1v8  "IO8_FT 100MHz low speed @ 1.8V pulldown"
io8_100m_ft_hs_3v3  "IO8_FT 100MHz high speed @ 3.3V"
io8_100m_ft_hs_pu_3v3  "IO8_FT 100MHz high speed @ 3.3V pullup"
io8_100m_ft_hs_pd_3v3  "IO8_FT 100MHz high speed @ 3.3V pulldown"
io8_100m_ft_fs_3v3  "IO8_FT 100MHz fast speed @ 3.3V"
io8_100m_ft_fs_pu_3v3  "IO8_FT 100MHz fast speed @ 3.3V pullup"
io8_100m_ft_fs_pd_3v3  "IO8_FT 100MHz fast speed @ 3.3V pulldown"
io8_100m_ft_ms_3v3  "IO8_FT 100MHz med speed @ 3.3V"
io8_100m_ft_ms_pu_3v3  "IO8_FT 100MHz med speed @ 3.3V pullup"
io8_100m_ft_ms_pd_3v3  "IO8_FT 100MHz med speed @ 3.3V pulldown"
io8_100m_ft_ls_3v3  "IO8_FT 100MHz low speed @ 3.3V"
io8_100m_ft_ls_pu_3v3  "IO8_FT 100MHz low speed @ 3.3V pullup"
io8_100m_ft_ls_pd_3v3  "IO8_FT 100MHz low speed @ 3.3V pulldown"
io8usb_id_nopu  "IOUSB ID @ 3.3V"
io8usb_id_pu  "IOUSB ID @ 3.3V pullup"
[Model Selector] io8_100m_usb_vbus_ft
io8_100m_ft_hs_1v2  "IO8_FT 100MHz high speed @ 1.2V"
io8_100m_ft_hs_pu_1v2  "IO8_FT 100MHz high speed @ 1.2V pullup"
io8_100m_ft_hs_pd_1v2  "IO8_FT 100MHz high speed @ 1.2V pulldown"
io8_100m_ft_fs_1v2  "IO8_FT 100MHz fast speed @ 1.2V"
io8_100m_ft_fs_pu_1v2  "IO8_FT 100MHz fast speed @ 1.2V pullup"
io8_100m_ft_fs_pd_1v2  "IO8_FT 100MHz fast speed @ 1.2V pulldown"
io8_100m_ft_ms_1v2  "IO8_FT 100MHz med speed @ 1.2V"
io8_100m_ft_ms_pu_1v2  "IO8_FT 100MHz med speed @ 1.2V pullup"
io8_100m_ft_ms_pd_1v2  "IO8_FT 100MHz med speed @ 1.2V pulldown"
io8_100m_ft_ls_1v2  "IO8_FT 100MHz low speed @ 1.2V"
io8_100m_ft_ls_pu_1v2  "IO8_FT 100MHz low speed @ 1.2V pullup"
io8_100m_ft_ls_pd_1v2  "IO8_FT 100MHz low speed @ 1.2V pulldown"
io8_100m_ft_hs_1v8  "IO8_FT 100MHz high speed @ 1.8V"
io8_100m_ft_hs_pu_1v8  "IO8_FT 100MHz high speed @ 1.8V pullup"
io8_100m_ft_hs_pd_1v8  "IO8_FT 100MHz high speed @ 1.8V pulldown"
io8_100m_ft_fs_1v8  "IO8_FT 100MHz fast speed @ 1.8V"
io8_100m_ft_fs_pu_1v8  "IO8_FT 100MHz fast speed @ 1.8V pullup"
io8_100m_ft_fs_pd_1v8  "IO8_FT 100MHz fast speed @ 1.8V pulldown"
io8_100m_ft_ms_1v8  "IO8_FT 100MHz med speed @ 1.8V"
io8_100m_ft_ms_pu_1v8  "IO8_FT 100MHz med speed @ 1.8V pullup"
io8_100m_ft_ms_pd_1v8  "IO8_FT 100MHz med speed @ 1.8V pulldown"
io8_100m_ft_ls_1v8  "IO8_FT 100MHz low speed @ 1.8V"
io8_100m_ft_ls_pu_1v8  "IO8_FT 100MHz low speed @ 1.8V pullup"
io8_100m_ft_ls_pd_1v8  "IO8_FT 100MHz low speed @ 1.8V pulldown"
io8_100m_ft_hs_3v3  "IO8_FT 100MHz high speed @ 3.3V"
io8_100m_ft_hs_pu_3v3  "IO8_FT 100MHz high speed @ 3.3V pullup"
io8_100m_ft_hs_pd_3v3  "IO8_FT 100MHz high speed @ 3.3V pulldown"
io8_100m_ft_fs_3v3  "IO8_FT 100MHz fast speed @ 3.3V"
io8_100m_ft_fs_pu_3v3  "IO8_FT 100MHz fast speed @ 3.3V pullup"
io8_100m_ft_fs_pd_3v3  "IO8_FT 100MHz fast speed @ 3.3V pulldown"
io8_100m_ft_ms_3v3  "IO8_FT 100MHz med speed @ 3.3V"
io8_100m_ft_ms_pu_3v3  "IO8_FT 100MHz med speed @ 3.3V pullup"
io8_100m_ft_ms_pd_3v3  "IO8_FT 100MHz med speed @ 3.3V pulldown"
io8_100m_ft_ls_3v3  "IO8_FT 100MHz low speed @ 3.3V"
io8_100m_ft_ls_pu_3v3  "IO8_FT 100MHz low speed @ 3.3V pullup"
io8_100m_ft_ls_pd_3v3  "IO8_FT 100MHz low speed @ 3.3V pulldown"
io8usb_adp "IOUSB ADP @ 3.3V"
io8usb_vbus "IOUSB VBUS @ 3.3V"
[Model Selector] io8_usb_ft
io8_100m_ft_hs_1v2  "IO8_FT 100MHz high speed @ 1.2V"
io8_100m_ft_hs_pu_1v2  "IO8_FT 100MHz high speed @ 1.2V pullup"
io8_100m_ft_hs_pd_1v2  "IO8_FT 100MHz high speed @ 1.2V pulldown"
io8_100m_ft_fs_1v2  "IO8_FT 100MHz fast speed @ 1.2V"
io8_100m_ft_fs_pu_1v2  "IO8_FT 100MHz fast speed @ 1.2V pullup"
io8_100m_ft_fs_pd_1v2  "IO8_FT 100MHz fast speed @ 1.2V pulldown"
io8_100m_ft_ms_1v2  "IO8_FT 100MHz med speed @ 1.2V"
io8_100m_ft_ms_pu_1v2  "IO8_FT 100MHz med speed @ 1.2V pullup"
io8_100m_ft_ms_pd_1v2  "IO8_FT 100MHz med speed @ 1.2V pulldown"
io8_100m_ft_ls_1v2  "IO8_FT 100MHz low speed @ 1.2V"
io8_100m_ft_ls_pu_1v2  "IO8_FT 100MHz low speed @ 1.2V pullup"
io8_100m_ft_ls_pd_1v2  "IO8_FT 100MHz low speed @ 1.2V pulldown"
io8_100m_ft_hs_1v8  "IO8_FT 100MHz high speed @ 1.8V"
io8_100m_ft_hs_pu_1v8  "IO8_FT 100MHz high speed @ 1.8V pullup"
io8_100m_ft_hs_pd_1v8  "IO8_FT 100MHz high speed @ 1.8V pulldown"
io8_100m_ft_fs_1v8  "IO8_FT 100MHz fast speed @ 1.8V"
io8_100m_ft_fs_pu_1v8  "IO8_FT 100MHz fast speed @ 1.8V pullup"
io8_100m_ft_fs_pd_1v8  "IO8_FT 100MHz fast speed @ 1.8V pulldown"
io8_100m_ft_ms_1v8  "IO8_FT 100MHz med speed @ 1.8V"
io8_100m_ft_ms_pu_1v8  "IO8_FT 100MHz med speed @ 1.8V pullup"
io8_100m_ft_ms_pd_1v8  "IO8_FT 100MHz med speed @ 1.8V pulldown"
io8_100m_ft_ls_1v8  "IO8_FT 100MHz low speed @ 1.8V"
io8_100m_ft_ls_pu_1v8  "IO8_FT 100MHz low speed @ 1.8V pullup"
io8_100m_ft_ls_pd_1v8  "IO8_FT 100MHz low speed @ 1.8V pulldown"
io8_100m_ft_hs_3v3  "IO8_FT 100MHz high speed @ 3.3V"
io8_100m_ft_hs_pu_3v3  "IO8_FT 100MHz high speed @ 3.3V pullup"
io8_100m_ft_hs_pd_3v3  "IO8_FT 100MHz high speed @ 3.3V pulldown"
io8_100m_ft_fs_3v3  "IO8_FT 100MHz fast speed @ 3.3V"
io8_100m_ft_fs_pu_3v3  "IO8_FT 100MHz fast speed @ 3.3V pullup"
io8_100m_ft_fs_pd_3v3  "IO8_FT 100MHz fast speed @ 3.3V pulldown"
io8_100m_ft_ms_3v3  "IO8_FT 100MHz med speed @ 3.3V"
io8_100m_ft_ms_pu_3v3  "IO8_FT 100MHz med speed @ 3.3V pullup"
io8_100m_ft_ms_pd_3v3  "IO8_FT 100MHz med speed @ 3.3V pulldown"
io8_100m_ft_ls_3v3  "IO8_FT 100MHz low speed @ 3.3V"
io8_100m_ft_ls_pu_3v3  "IO8_FT 100MHz low speed @ 3.3V pullup"
io8_100m_ft_ls_pd_3v3  "IO8_FT 100MHz low speed @ 3.3V pulldown"
io8_usb_fs_3v3  "IOUSB fast speed @ 3.3V"
io8_usb_fs_pu1_3v3  "IO8USB fast speed @ 3.3V pullup1"
io8_usb_fs_pd1_3v3  "IOUSB fast speed @ 3.3V pulldown1"
io8_usb_ls_3v3  "IOUSB low speed @ 3.3V"
io8_usb_ls_pu1_3v3  "IOUSB low speed @ 3.3V pullup1"
io8_usb_ls_pd1_3v3  "IOUSB low speed @ 3.3V pulldown1"
io8_usb_fs_pu2_3v3  "IOUSB fast speed @ 3.3V pullup2"
io8_usb_fs_pd2_3v3  "IOUSB fast speed @ 3.3V pulldown2"
io8_usb_ls_pu2_3v3  "IOUSB low speed @ 3.3V pullup2"
io8_usb_ls_pd2_3v3  "IOUSB low speed @ 3.3V pulldown2"
[Model Selector] io8_100m_i2c_ft
io8_100m_ft_hs_1v2  "IO8_FT 100MHz high speed @ 1.2V"
io8_100m_ft_hs_pu_1v2  "IO8_FT 100MHz high speed @ 1.2V pullup"
io8_100m_ft_hs_pd_1v2  "IO8_FT 100MHz high speed @ 1.2V pulldown"
io8_100m_ft_fs_1v2  "IO8_FT 100MHz fast speed @ 1.2V"
io8_100m_ft_fs_pu_1v2  "IO8_FT 100MHz fast speed @ 1.2V pullup"
io8_100m_ft_fs_pd_1v2  "IO8_FT 100MHz fast speed @ 1.2V pulldown"
io8_100m_ft_ms_1v2  "IO8_FT 100MHz med speed @ 1.2V"
io8_100m_ft_ms_pu_1v2  "IO8_FT 100MHz med speed @ 1.2V pullup"
io8_100m_ft_ms_pd_1v2  "IO8_FT 100MHz med speed @ 1.2V pulldown"
io8_100m_ft_ls_1v2  "IO8_FT 100MHz low speed @ 1.2V"
io8_100m_ft_ls_pu_1v2  "IO8_FT 100MHz low speed @ 1.2V pullup"
io8_100m_ft_ls_pd_1v2  "IO8_FT 100MHz low speed @ 1.2V pulldown"
io8_100m_ft_hs_1v8  "IO8_FT 100MHz high speed @ 1.8V"
io8_100m_ft_hs_pu_1v8  "IO8_FT 100MHz high speed @ 1.8V pullup"
io8_100m_ft_hs_pd_1v8  "IO8_FT 100MHz high speed @ 1.8V pulldown"
io8_100m_ft_fs_1v8  "IO8_FT 100MHz fast speed @ 1.8V"
io8_100m_ft_fs_pu_1v8  "IO8_FT 100MHz fast speed @ 1.8V pullup"
io8_100m_ft_fs_pd_1v8  "IO8_FT 100MHz fast speed @ 1.8V pulldown"
io8_100m_ft_ms_1v8  "IO8_FT 100MHz med speed @ 1.8V"
io8_100m_ft_ms_pu_1v8  "IO8_FT 100MHz med speed @ 1.8V pullup"
io8_100m_ft_ms_pd_1v8  "IO8_FT 100MHz med speed @ 1.8V pulldown"
io8_100m_ft_ls_1v8  "IO8_FT 100MHz low speed @ 1.8V"
io8_100m_ft_ls_pu_1v8  "IO8_FT 100MHz low speed @ 1.8V pullup"
io8_100m_ft_ls_pd_1v8  "IO8_FT 100MHz low speed @ 1.8V pulldown"
io8_100m_ft_hs_3v3  "IO8_FT 100MHz high speed @ 3.3V"
io8_100m_ft_hs_pu_3v3  "IO8_FT 100MHz high speed @ 3.3V pullup"
io8_100m_ft_hs_pd_3v3  "IO8_FT 100MHz high speed @ 3.3V pulldown"
io8_100m_ft_fs_3v3  "IO8_FT 100MHz fast speed @ 3.3V"
io8_100m_ft_fs_pu_3v3  "IO8_FT 100MHz fast speed @ 3.3V pullup"
io8_100m_ft_fs_pd_3v3  "IO8_FT 100MHz fast speed @ 3.3V pulldown"
io8_100m_ft_ms_3v3  "IO8_FT 100MHz med speed @ 3.3V"
io8_100m_ft_ms_pu_3v3  "IO8_FT 100MHz med speed @ 3.3V pullup"
io8_100m_ft_ms_pd_3v3  "IO8_FT 100MHz med speed @ 3.3V pulldown"
io8_100m_ft_ls_3v3  "IO8_FT 100MHz low speed @ 3.3V"
io8_100m_ft_ls_pu_3v3  "IO8_FT 100MHz low speed @ 3.3V pullup"
io8_100m_ft_ls_pd_3v3  "IO8_FT 100MHz low speed @ 3.3V pulldown"
io8_100m_i2c_ft_1v2  "IO8_FT 100MHz I2C @ 1.2V"
io8_100m_i2c_ft_pu_1v2  "IO8_FT 100MHz I2C @ 1.2V pullup"
io8_100m_i2c_ft_pd_1v2  "IO8_FT 100MHz I2C @ 1.2V pulldown"
io8_100m_i2c_ft_1v8  "IO8_FT 100MHz I2C @ 1.8V"
io8_100m_i2c_ft_pu_1v8  "IO8_FT 100MHz I2C @ 1.8V pullup"
io8_100m_i2c_ft_pd_1v8  "IO8_FT 100MHz I2C @ 1,8V pulldown"
io8_100m_i2c_ft_3v3  "IO8_FT 100MHz I2C @ 3.3V"
io8_100m_i2c_ft_pu_3v3  "IO8_FT 100MHz I2C HSLV @ 3.3V pullup"
io8_100m_i2c_ft_pd_3v3  "IO8_FT 100MHz I2C @ 3.3V pulldown"
[Model Selector] io8_166m_hslv_i2c_ft
io8_166m_ft_hs_1v2  "IO8_FT 166MHz high speed @ 1.2V"
io8_166m_ft_hs_pu_1v2  "IO8_FT 166MHz high speed @ 1.2V pullup"
io8_166m_ft_hs_pd_1v2  "IO8_FT 166MHz high speed @ 1.2V pulldown"
io8_166m_ft_fs_1v2  "IO8_FT 166MHz fast speed @ 1.2V"
io8_166m_ft_fs_pu_1v2  "IO8_FT 166MHz fast speed @ 1.2V pullup"
io8_166m_ft_fs_pd_1v2  "IO8_FT 166MHz fast speed @ 1.2V pulldown"
io8_166m_ft_ms_1v2  "IO8_FT 166MHz med speed @ 1.2V"
io8_166m_ft_ms_pu_1v2  "IO8_FT 166MHz med speed @ 1.2V pullup"
io8_166m_ft_ms_pd_1v2  "IO8_FT 166MHz med speed @ 1.2V pulldown"
io8_166m_ft_ls_1v2  "IO8_FT 166MHz low speed @ 1.2V"
io8_166m_ft_ls_pu_1v2  "IO8_FT 166MHz low speed @ 1.2V pullup"
io8_166m_ft_ls_pd_1v2  "IO8_FT 166MHz low speed @ 1.2V pulldown"
io8_166m_ft_hs_1v8  "IO8_FT 166MHz high speed @ 1.8V"
io8_166m_ft_hs_pu_1v8  "IO8_FT 166MHz high speed @ 1.8V pullup"
io8_166m_ft_hs_pd_1v8  "IO8_FT 166MHz high speed @ 1.8V pulldown"
io8_166m_ft_fs_1v8  "IO8_FT 166MHz fast speed @ 1.8V"
io8_166m_ft_fs_pu_1v8  "IO8_FT 166MHz fast speed @ 1.8V pullup"
io8_166m_ft_fs_pd_1v8  "IO8_FT 166MHz fast speed @ 1.8V pulldown"
io8_166m_ft_ms_1v8  "IO8_FT 166MHz med speed @ 1.8V"
io8_166m_ft_ms_pu_1v8  "IO8_FT 166MHz med speed @ 1.8V pullup"
io8_166m_ft_ms_pd_1v8  "IO8_FT 166MHz med speed @ 1.8V pulldown"
io8_166m_ft_ls_1v8  "IO8_FT 166MHz low speed @ 1.8V"
io8_166m_ft_ls_pu_1v8  "IO8_FT 166MHz low speed @ 1.8V pullup"
io8_166m_ft_ls_pd_1v8  "IO8_FT 166MHz low speed @ 1.8V pulldown"
io8_166m_ft_hs_3v3  "IO8_FT 166MHz high speed @ 3.3V"
io8_166m_ft_hs_pu_3v3  "IO8_FT 166MHz high speed @ 3.3V pullup"
io8_166m_ft_hs_pd_3v3  "IO8_FT 166MHz high speed @ 3.3V pulldown"
io8_166m_ft_fs_3v3  "IO8_FT 166MHz fast speed @ 3.3V"
io8_166m_ft_fs_pu_3v3  "IO8_FT 166MHz fast speed @ 3.3V pullup"
io8_166m_ft_fs_pd_3v3  "IO8_FT 166MHz fast speed @ 3.3V pulldown"
io8_166m_ft_ms_3v3  "IO8_FT 166MHz med speed @ 3.3V"
io8_166m_ft_ms_pu_3v3  "IO8_FT 166MHz med speed @ 3.3V pullup"
io8_166m_ft_ms_pd_3v3  "IO8_FT 166MHz med speed @ 3.3V pulldown"
io8_166m_ft_ls_3v3  "IO8_FT 166MHz low speed @ 3.3V"
io8_166m_ft_ls_pu_3v3  "IO8_FT 166MHz low speed @ 3.3V pullup"
io8_166m_ft_ls_pd_3v3  "IO8_FT 166MHz low speed @ 3.3V pulldown"
io8_166m_hslv_ft_hs_1v2  "IO8_FT 166MHz HSLV high speed @ 1.2V"
io8_166m_hslv_ft_hs_pu_1v2  "IO8_FT 166MHz HSLV high speed @ 1.2V pullup"
io8_166m_hslv_ft_hs_pd_1v2  "IO8_FT 166MHz HSLV high speed @ 1.2V pulldown"
io8_166m_hslv_ft_fs_1v2  "IO8_FT 166MHz HSLV fast speed @ 1.2V"
io8_166m_hslv_ft_fs_pu_1v2  "IO8_FT 166MHz HSLV fast speed @ 1.2V pullup"
io8_166m_hslv_ft_fs_pd_1v2  "IO8_FT 166MHz HSLV fast speed @ 1.2V pulldown"
io8_166m_hslv_ft_ms_1v2  "IO8_FT 166MHz HSLV med speed @ 1.2V"
io8_166m_hslv_ft_ms_pu_1v2  "IO8_FT 166MHz HSLV med speed @ 1.2V pullup"
io8_166m_hslv_ft_ms_pd_1v2  "IO8_FT 166MHz HSLV med speed @ 1.2V pulldown"
io8_166m_hslv_ft_ls_1v2  "IO8_FT 166MHz HSLV low speed @ 1.2V"
io8_166m_hslv_ft_ls_pu_1v2  "IO8_FT 166MHz HSLV low speed @ 1.2V pullup"
io8_166m_hslv_ft_ls_pd_1v2  "IO8_FT 166MHz HSLV low speed @ 1.2V pulldown"
io8_166m_hslv_ft_hs_1v8  "IO8_FT 166MHz HSLV high speed @ 1.8V"
io8_166m_hslv_ft_hs_pu_1v8  "IO8_FT 166MHz HSLV high speed @ 1.8V pullup"
io8_166m_hslv_ft_hs_pd_1v8  "IO8_FT 166MHz HSLV high speed @ 1.8V pulldown"
io8_166m_hslv_ft_fs_1v8  "IO8_FT 166MHz HSLV fast speed @ 1.8V"
io8_166m_hslv_ft_fs_pu_1v8  "IO8_FT 166MHz HSLV fast speed @ 1.8V pullup"
io8_166m_hslv_ft_fs_pd_1v8  "IO8_FT 166MHz HSLV fast speed @ 1.8V pulldown"
io8_166m_hslv_ft_ms_1v8  "IO8_FT 166MHz HSLV med speed @ 1.8V"
io8_166m_hslv_ft_ms_pu_1v8  "IO8_FT 166MHz HSLV med speed @ 1.8V pullup"
io8_166m_hslv_ft_ms_pd_1v8  "IO8_FT 166MHz HSLV med speed @ 1.8V pulldown"
io8_166m_hslv_ft_ls_1v8  "IO8_FT 166MHz HSLV low speed @ 1.8V"
io8_166m_hslv_ft_ls_pu_1v8  "IO8_FT 166MHz HSLV low speed @ 1.8V pullup"
io8_166m_hslv_ft_ls_pd_1v8  "IO8_FT 166MHz HSLV low speed @ 1.8V pulldown"
io8_166m_hslv_ft_hs_2v5  "IO8_FT 166MHz HSLV high speed @ 2.5V"
io8_166m_hslv_ft_hs_pu_2v5  "IO8_FT 166MHz HSLV high speed @ 2.5V pullup"
io8_166m_hslv_ft_hs_pd_2v5  "IO8_FT 166MHz HSLV high speed @ 2.5V pulldown"
io8_166m_hslv_ft_fs_2v5  "IO8_FT 166MHz HSLV fast speed @ 2.5V"
io8_166m_hslv_ft_fs_pu_2v5  "IO8_FT 166MHz HSLV fast speed @ 2.5V pullup"
io8_166m_hslv_ft_fs_pd_2v5  "IO8_FT 166MHz HSLV fast speed @ 2.5V pulldown"
io8_166m_hslv_ft_ms_2v5  "IO8_FT 166MHz HSLV med speed @ 2.5V"
io8_166m_hslv_ft_ms_pu_2v5  "IO8_FT 166MHz HSLV med speed @ 2.5V pullup"
io8_166m_hslv_ft_ms_pd_2v5  "IO8_FT 166MHz HSLV med speed @ 2.5V pulldown"
io8_166m_hslv_ft_ls_2v5  "IO8_FT 166MHz HSLV low speed @ 2.5V"
io8_166m_hslv_ft_ls_pu_2v5  "IO8_FT 166MHz HSLV low speed @ 2.5V pullup"
io8_166m_hslv_ft_ls_pd_2v5  "IO8_FT 166MHz HSLV low speed @ 2.5V pulldown"
io8_166m_i2c_ft_1v2  "IO8_FT 166MHz I2C @ 1.2V"
io8_166m_i2c_ft_pu_1v2  "IO8_FT 166MHz I2C @ 1.2V pullup"
io8_166m_i2c_ft_pd_1v2  "IO8_FT 166MHz I2C @ 1.2V pulldown"
io8_166m_i2c_ft_1v8  "IO8_FT 166MHz I2C @ 1.8V"
io8_166m_i2c_ft_pu_1v8  "IO8_FT 166MHz I2C @ 1.8V pullup"
io8_166m_i2c_ft_pd_1v8  "IO8_FT 166MHz I2C @ 1,8V pulldown"
io8_166m_i2c_ft_3v3  "IO8_FT 166MHz I2C @ 3.3V"
io8_166m_i2c_ft_pu_3v3  "IO8_FT 166MHz I2C HSLV @ 3.3V pullup"
io8_166m_i2c_ft_pd_3v3  "IO8_FT 166MHz I2C @ 3.3V pulldown"
| Models and submodels in the file (212): io8_100m_ft_hs_1v2 (I/O), io8_100m_ft_hs_pu_1v2 (I/O), io8_100m_ft_hs_pd_1v2 (I/O), io8_100m_ft_fs_1v2 (I/O), io8_100m_ft_fs_pu_1v2 (I/O), io8_100m_ft_fs_pd_1v2 (I/O), io8_100m_ft_ms_1v2 (I/O), io8_100m_ft_ms_pu_1v2 (I/O), io8_100m_ft_ms_pd_1v2 (I/O), io8_100m_ft_ls_1v2 (I/O), io8_100m_ft_ls_pu_1v2 (I/O), io8_100m_ft_ls_pd_1v2 (I/O), io8_100m_ft_hs_1v8 (I/O), io8_100m_ft_hs_pu_1v8 (I/O), io8_100m_ft_hs_pd_1v8 (I/O), io8_100m_ft_fs_1v8 (I/O), io8_100m_ft_fs_pu_1v8 (I/O), io8_100m_ft_fs_pd_1v8 (I/O), io8_100m_ft_ms_1v8 (I/O), io8_100m_ft_ms_pu_1v8 (I/O), io8_100m_ft_ms_pd_1v8 (I/O), io8_100m_ft_ls_1v8 (I/O), io8_100m_ft_ls_pu_1v8 (I/O), io8_100m_ft_ls_pd_1v8 (I/O), io8_100m_ft_hs_3v3 (I/O), io8_100m_ft_hs_pu_3v3 (I/O), io8_100m_ft_hs_pd_3v3 (I/O), io8_100m_ft_fs_3v3 (I/O), io8_100m_ft_fs_pu_3v3 (I/O), io8_100m_ft_fs_pd_3v3 (I/O), io8_100m_ft_ms_3v3 (I/O), io8_100m_ft_ms_pu_3v3 (I/O), io8_100m_ft_ms_pd_3v3 (I/O), io8_100m_ft_ls_3v3 (I/O), io8_100m_ft_ls_pu_3v3 (I/O), io8_100m_ft_ls_pd_3v3 (I/O), io8_100m_hslv_ft_hs_1v2 (I/O), io8_100m_hslv_ft_hs_pu_1v2 (I/O), io8_100m_hslv_ft_hs_pd_1v2 (I/O), io8_100m_hslv_ft_fs_1v2 (I/O), io8_100m_hslv_ft_fs_pu_1v2 (I/O), io8_100m_hslv_ft_fs_pd_1v2 (I/O), io8_100m_hslv_ft_ms_1v2 (I/O), io8_100m_hslv_ft_ms_pu_1v2 (I/O), io8_100m_hslv_ft_ms_pd_1v2 (I/O), io8_100m_hslv_ft_ls_1v2 (I/O), io8_100m_hslv_ft_ls_pu_1v2 (I/O), io8_100m_hslv_ft_ls_pd_1v2 (I/O), io8_100m_hslv_ft_hs_1v8 (I/O), io8_100m_hslv_ft_hs_pu_1v8 (I/O), io8_100m_hslv_ft_hs_pd_1v8 (I/O), io8_100m_hslv_ft_fs_1v8 (I/O), io8_100m_hslv_ft_fs_pu_1v8 (I/O), io8_100m_hslv_ft_fs_pd_1v8 (I/O), io8_100m_hslv_ft_ms_1v8 (I/O), io8_100m_hslv_ft_ms_pu_1v8 (I/O), io8_100m_hslv_ft_ms_pd_1v8 (I/O), io8_100m_hslv_ft_ls_1v8 (I/O), io8_100m_hslv_ft_ls_pu_1v8 (I/O), io8_100m_hslv_ft_ls_pd_1v8 (I/O), io8_100m_hslv_ft_hs_2v5 (I/O), io8_100m_hslv_ft_hs_pu_2v5 (I/O), io8_100m_hslv_ft_hs_pd_2v5 (I/O), io8_100m_hslv_ft_fs_2v5 (I/O), io8_100m_hslv_ft_fs_pu_2v5 (I/O), io8_100m_hslv_ft_fs_pd_2v5 (I/O), io8_100m_hslv_ft_ms_2v5 (I/O), io8_100m_hslv_ft_ms_pu_2v5 (I/O), io8_100m_hslv_ft_ms_pd_2v5 (I/O), io8_100m_hslv_ft_ls_2v5 (I/O), io8_100m_hslv_ft_ls_pu_2v5 (I/O), io8_100m_hslv_ft_ls_pd_2v5 (I/O), io8_166m_ft_hs_1v2 (I/O), io8_166m_ft_hs_pu_1v2 (I/O), io8_166m_ft_hs_pd_1v2 (I/O), io8_166m_ft_fs_1v2 (I/O), io8_166m_ft_fs_pu_1v2 (I/O), io8_166m_ft_fs_pd_1v2 (I/O), io8_166m_ft_ms_1v2 (I/O), io8_166m_ft_ms_pu_1v2 (I/O)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
